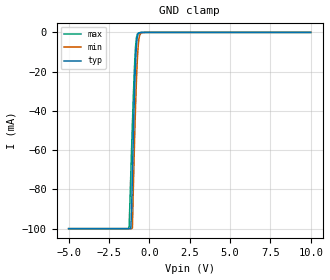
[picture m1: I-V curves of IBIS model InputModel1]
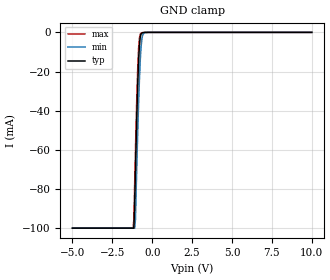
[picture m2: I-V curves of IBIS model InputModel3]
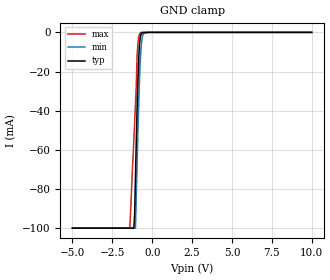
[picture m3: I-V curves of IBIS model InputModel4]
[IBIS Ver]   2.1
[File name]   e_032sa5.ibs   | e_= TSOP, f032sa= abbr chip name, 5= 5 V Vcc
[File Rev]   2.00
[Date]   26-February-96
[Source]   File generated from lab measurements at Intel Corporation
[Notes]   Rev 2.00   All data from actual measurements performed in a lab.
[Disclaimer] INTEL DEVELOPER'S SOFTWARE LICENSE AGREEMENT
| BY USING THIS SOFTWARE, YOU ARE AGREEING TO BE BOUND
| BY THE TERMS OF THIS AGREEMENT.  DO NOT USE THE SOFTWARE
| UNTIL YOU HAVE CAREFULLY READ AND AGREED TO THE FOLLOWING
| TERMS AND CONDITIONS.  IF YOU DO NOT AGREE TO THE TERMS
| OF THIS AGREEMENT, PROMPTLY RETURN THE SOFTWARE PACKAGE
| AND ANY ACCOMPANYING ITEMS.
| IF YOU USE THIS SOFTWARE, YOU WILL BE BOUND BY THE TERMS
| OF THIS AGREEMENT
| LICENSE: Intel Corporation ("Intel") grants you the non-exclusive right
| to use the enclosed software program ("Software").  You will not use,
| copy, modify, rent, sell or transfer the Software or any portion
| thereof, except as provided in this Agreement.
| System OEM Developers may:
| 1.   Copy the Software for support, backup or archival purposes;
| 2.   Install, use, or distribute Intel owned Software in object code
|   only;
| 3.   Modify and/or use Software source code that Intel directly makes
|   available to you as an OEM Developer;
| 4.   Install, use, modify, distribute, and/or make or have made
|   derivatives ("Derivatives") of Intel owned Software under the
|   terms and conditions in this Agreement, ONLY if you are a System
|   OEM Developer and NOT an end-user.
| RESTRICTIONS:
| YOU WILL NOT:
| 1.   Copy the Software, in whole or in part, except as provided for
|   in this Agreement;
| 2.   Decompile or reverse engineer any Software provided in object
|   code format;
| 3.   Distribute any Software or Derivative code to any end-users,
|   unless approved by Intel in a prior writing.
| TRANSFER: You may transfer the Software to another OEM
| Developer if thereceiving party agrees to the terms of this
| Agreement at the sole risk of any receiving party.
| OWNERSHIP AND COPYRIGHT OF SOFTWARE:
| Title to the Software and all copies thereof remain with Intel
| or its vendors.  The Software iscopyrighted and is protected by
| United States and international copyright laws.  You will not
| remove the copyright notice from the Software.  You agree to
| prevent any unauthorized copying of the Software.
| DERIVATIVE WORK: OEM Developers that make or have made
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[Copyright]   Copyright 1996, Intel Corporation, All Rights Reserved
[Component]   E28F032SA   | 56-lead TSOP package, 28F032SA
[Manufacturer]  Intel   | FlashFile(tm) Memory
|   | operating in 5.0 V Vcc range
|********************Pin and Package Definitions*********************
[Package]
|The following values apply for the Copper leadframe.
|Variable   typ   min   max
R_pkg   48m   41m   54m
L_pkg   4.92nH   4.44nH   5.39nH
C_pkg   0.48pF   0.45pF   0.50pF
|The following values apply for the Alloy-42 leadframe.
|Variable   typ   min   max
|R_pkg   195m   180m   210m
|L_pkg   4.92nH   4.44nH   5.39nH
|C_pkg   0.48pF   0.45pF   0.50pF
|***********************Pin Defintions*************************************
[Pin] signal_name   model_name   R_pin   L_pin   C_pin
  1   3/5#   InputModel1
  2   CE1#   InputModel5
  3   CE2#   InputModel6
  4   A20   InputModel3
  5   A19   InputModel3
  6   A18   InputModel1
  7   A17   InputModel1
  8   A16   InputModel1
  9   VCC   POWER
 10   A15   InputModel1
 11   A14   InputModel3
 12   A13   InputModel1
 13   A12   InputModel1
 14   CE0#   InputModel1
 15   VPP   POWER
 16   RP#   InputModel4
 17   A11   InputModel1
 18   A10   InputModel1
 19   A9   InputModel1
 20   A8   InputModel1
 21   GND   GND
 22   A7   InputModel1
 23   A6   InputModel1
 24   A5   InputModel1
 25   A4   InputModel1
 26   A3   InputModel1
 27   A2   InputModel1
 28   A1   InputModel1
 29   NC   InputModel2
 30   NC   InputModel2
 31   BYTE#   InputModel1
 32   A0   InputModel1
 33   DQ0   InputOutput
 34   DQ8   InputOutput
 35   DQ1   InputOutput
 36   DQ9   InputOutput
 37   VCC   POWER
 38   DQ2   InputOutput
 39   DQ10   InputOutput
 40   DQ3   InputOutput
 41   DQ11   InputOutput
 42   GND   GND
 43   VCC   POWER
 44   DQ4   InputOutput
 45   DQ12   InputOutput
 46   DQ5   InputOutput
 47   DQ13   InputOutput
 48   GND   GND
 49   DQ6   InputOutput
 50   DQ14   InputOutput
 51   DQ7   InputOutput
 52   DQ15   InputOutput
 53   RY/BY#   OpenDrainOutput
 54   OE#   InputModel1
 55   WE#   InputModel4
 56   WP#   InputModel1
|*************************Input Model 2***************************
[Model]   InputModel2
Model_type   Input
|   For NC (Pins 29 & 30)
Vinl = 0.8V
Vinh = 2.0V
| Variable   typ   min   max
C_comp   5.61p   NA   7.6p
[Voltage Range]   5.0V   4.5V   5.5V
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| Models and submodels in the file (8): InputModel1 (Input), InputModel2 (Input), InputModel3 (Input), InputModel4 (Input), InputModel5 (Input), InputModel6 (Input), InputOutput (I/O), OpenDrainOutput (Open_drain)
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|**********************Input Model 1 *******************************
[Model]   InputModel1
Model_type   Input
|   For pin1(3/5#), CE0#, OE#, WP#, BYTE#, A[18:15], A[13:0]
Vinl = 0.8V
Vinh = 2.0V
|Variable   typ   min   max
C_comp   5.61p   NA   7.6p
[Voltage Range]   5.0V   4.5V   5.5V
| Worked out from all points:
|   GND clamp passes 1 mA (typ) near -0.70 V on its own axis
[GND_clamp]
|Voltage I(typ)   I(min)   I(max)
-5V       -100mA     -100mA     -100mA
-1.3V     -100mA     -100mA     -100mA
-1.25V    -100mA     -100mA     -98.91mA
-1.15V    -100mA     -100mA     -72.51mA
-1.1V     -90.9mA    -100mA     -59.43mA
-1.05V    -72.64mA   -99.73mA   -46.73mA
-950mV    -39.54mA   -65.95mA   -23.49mA
-850mV    -14.56mA   -36.83mA   -6.92mA
-700mV    -889.4uA   -7.755mA   -445.6uA
-600mV    -189.1uA   -1.422mA   -133.9uA
-250mV    0A         0A         0A
10V       0A         0A         0A
[POWER_clamp]
| Input buffer circuits of this product do not intrinsically
| require a [POWER_clamp] definition.  This zero current
| [POWER_clamp] is provided for compatibility with some ibis
| parsers.
|   Voltage  I(typ)   I(min)   I(max)
-5V       0A         0A         0A
-4.75V    0A         0A         0A
9.75V     0A         0A         0A
10V       0A         0A         0A
|***************************Input Model 3****************************
[Model]   InputModel3
Model_type   Input
|   for A[20], A[19], A[14]
Vinl = 0.8V
Vinh = 2.0V
| Variable   typ   min   max
C_comp   5.61p   NA   7.6p
[Voltage Range]   5.0V   4.5V   5.5V
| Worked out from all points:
|   GND clamp passes 1 mA (typ) near -0.70 V on its own axis
[GND_clamp]
|Voltage I(typ)   I(min)   I(max)
-5V       -100mA     -100mA     -100mA
-1.2V     -100mA     -100mA     -100mA
-1.15V    -100mA     -100mA     -95.76mA
-1.1V     -88mA      -100mA     -77.62mA
-1.05V    -70.66mA   -95.63mA   -60.12mA
-950mV    -38.55mA   -63.37mA   -28.82mA
-900mV    -24.89mA   -48.71mA   -16.47mA
-800mV    -6.521mA   -23.8mA    -2.802mA
-700mV    -863.8uA   -7.637mA   -429.7uA
-600mV    -177.6uA   -1.406mA   -126.2uA
-250mV    0A         0A         0A
10V       0A         0A         0A
[POWER_clamp]
| Input buffer circuits of this product do not intrinsically
| require a [POWER_clamp] definition.  This zero current
| [POWER_clamp] is provided for compatibility with some ibis
| parsers.
|   Voltage  I(typ)   I(min)   I(max)
-5V       0A         0A         0A
-4.75V    0A         0A         0A
9.75V     0A         0A         0A
10V       0A         0A         0A
|*************************Input Model 4*****************************
[Model]   InputModel4
Model_type   Input
|   For RP#, WE#
Vinl = 0.8V
Vinh = 2.0V
| Variable   typ   min   max
C_comp   5.61p   NA   7.6p
[Voltage Range]   5.0V   4.5V   5.5V
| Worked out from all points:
|   GND clamp passes 1 mA (typ) near -0.70 V on its own axis
[GND_clamp]
|Voltage I(typ)   I(min)   I(max)
-5V       -100mA     -100mA     -100mA
-1.4V     -100mA     -100mA     -100mA
-1.15V    -100mA     -100mA     -54.9mA
-1.1V     -93.14mA   -100mA     -45.76mA
-1.05V    -74.21mA   -100mA     -36.59mA
-1V       -56.45mA   -85.04mA   -27.72mA
-950mV    -39.9mA    -67.97mA   -12mA
-850mV    -14.42mA   -37.65mA   -2.593mA
-700mV    -868.6uA   -7.808mA   0A
-600mV    -186uA     -1.477mA   0A
-250mV    0A         0A         0A
10V       0A         0A         0A
[POWER_clamp]
| Input buffer circuits of this product do not intrinsically
| require a [POWER_clamp] definition.  This zero current
| [POWER_clamp] is provided for compatibility with some ibis
| parsers.
|   Voltage  I(typ)   I(min)   I(max)
-5V       0A         0A         0A
-4.75V    0A         0A         0A
9.75V     0A         0A         0A
10V       0A         0A         0A
